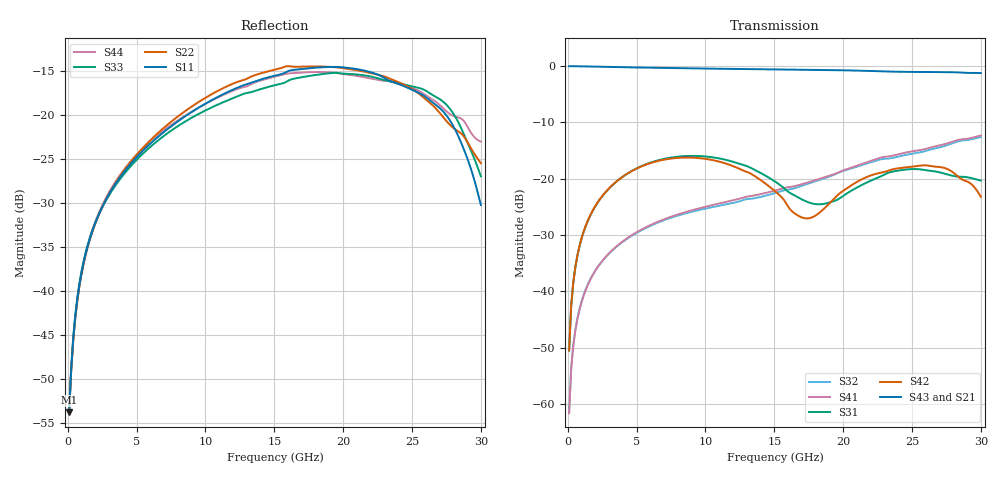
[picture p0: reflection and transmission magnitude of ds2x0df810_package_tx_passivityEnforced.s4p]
!Generated from:
! 1
! 2
! 3
! 4
!SystemSI_SerialLink Version: 17.1.6.09121.105558  006
!Computer Host Name: NAVEEN-DT
!TouchstoneFormatFlag = 1
!User Comments:
!  S-Parameters data
!  Freq  dbS11  angS11  dbS12  angS12  dbS13  angS13  dbS14  angS14
!  dbS21  angS21  dbS22  angS22  dbS23  angS23  dbS24  angS24
!  dbS31  angS31  dbS32  angS32  dbS33  angS33  dbS34  angS34
!  dbS41  angS41  dbS42  angS42  dbS43  angS43  dbS44  angS44
#	Hz	S	RI	R	50
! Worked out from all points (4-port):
!   200 points, 100 MHz to 30 GHz, reference 50 ohm
!   strongest paths, dB at 100 MHz, 7.613 GHz, 15.13 GHz, 22.64 GHz, 30 GHz:
!     S43: 0.0, -0.4, -0.6, -0.9, -1.2
!     S21: 0.0, -0.4, -0.6, -0.9, -1.3
!     S42: -50.5, -16.4, -22.4, -19.0, -23.2
!     S31: -50.5, -16.2, -20.6, -19.7, -20.3
!     S41: -61.7, -26.7, -22.1, -16.3, -12.3
!     S32: -61.5, -26.8, -22.5, -16.6, -12.6
!   lowest |S11| = -53.8 dB at 100 MHz (marker M1), VSWR 1.00, Z = 50.2 + j0.124 ohm
!   |S11| at or under -10 dB: start of sweep to end of sweep
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1e8  0.00161 0.00124  0.9978 -0.0192  0.000279 0.00297  -0.00015 -0.000812
     0.9978 -0.0192  0.00161 0.00119  -0.00015 -0.00083  0.000269 0.00298
     0.000279 0.00297  -0.00015 -0.00083  0.00159 0.00128  0.9979 -0.0189
     -0.00015 -0.000812  0.000269 0.00298  0.9979 -0.0189  0.00165 0.00121
1.151759e9  0.00411 0.0138  0.9697 -0.2166  0.00873 0.0325  -0.00289 -0.00866
            0.9697 -0.2166  0.0065 0.0126  -0.00306 -0.00875  0.00727 0.033
            0.00873 0.0325  -0.00306 -0.00875  0.00461 0.014  0.9706 -0.2127
            -0.00289 -0.00866  0.00727 0.033  0.9706 -0.2127  0.00615 0.0131
4.457286e9  0.0289 0.0423  0.6608 -0.716  0.0913 0.0675  -0.026 -0.0159
            0.6608 -0.716  0.0504 0.0147  -0.0258 -0.0154  0.0774 0.0828
            0.0913 0.0675  -0.0258 -0.0154  0.03 0.0396  0.6718 -0.7056
            -0.026 -0.0159  0.0774 0.0828  0.6718 -0.7056  0.0495 0.0188
1.016683e10  0.1115 0.0364  -0.2662 -0.9107  0.1334 -0.0825  -0.0506 0.0263
             -0.2662 -0.9107  0.0696 -0.1059  -0.0486 0.0253  0.1489 -0.00386
             0.1334 -0.0825  -0.0486 0.0253  0.1031 0.029  -0.2326 -0.9206
             -0.0506 0.0263  0.1489 -0.00386  -0.2326 -0.9206  0.0733 -0.091
1.677789e10  0.1442 -0.109  -0.9198 -0.0816  -0.0559 -0.0382  -0.00758 0.0875
             -0.9198 -0.0816  -0.1272 -0.1369  -0.0138 0.0836  0.0461 -0.00679
             -0.0559 -0.0382  -0.0138 0.0836  0.1369 -0.0863  -0.9177 -0.1391
             -0.00758 0.0875  0.0461 -0.00679  -0.9177 -0.1391  -0.1058 -0.1366
2.398995e10  -0.0375 -0.1447  -0.2879 0.8424  0.0843 0.0826  0.154 0.0582
             -0.2879 0.8424  -0.1394 0.063  0.1425 0.0661  0.1176 0.0382
             0.0843 0.0826  0.1425 0.0661  -0.00867 -0.1508  -0.3627 0.8133
             0.154 0.0582  0.1176 0.0382  -0.3627 0.8133  -0.1413 0.0495
3e10  -0.0253 -0.0172  0.6372 0.58  0.0934 -0.0231  0.1517 -0.1888
      0.6372 0.58  -0.0235 0.0474  0.166 -0.1666  0.0447 -0.0526
      0.0934 -0.0231  0.166 -0.1666  -0.0361 -0.0262  0.5611 0.6621
      0.1517 -0.1888  0.0447 -0.0526  0.5611 0.6621  -0.0387 0.0585
